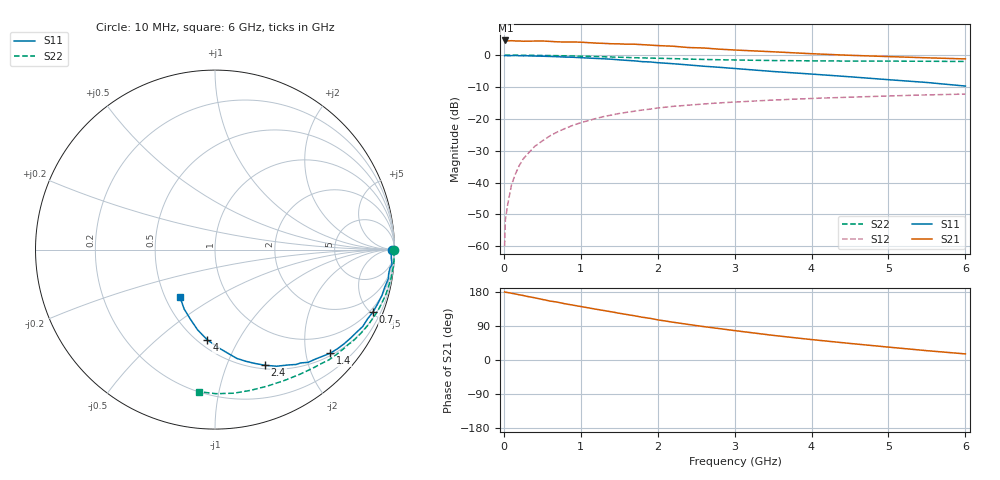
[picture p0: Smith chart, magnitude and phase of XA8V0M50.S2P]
! SIEMENS Discrete & RF Semiconductors
! BFY180
! Si NPN RF Bipolar Junction Transistor in MICRO-X
! VCE = 8 V  IC = 0.5 mA
! Common Emitter S-Parameters:  May  1997
# GHz  S  MA  R  50
!  f  S11  S21  S12  S22
! GHz  MAG  ANG  MAG  ANG  MAG  ANG  MAG  ANG
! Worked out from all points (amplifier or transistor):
!   36 points, 10 MHz to 6 GHz, reference 50 ohm
!   highest |S21| = 4.6 dB at 20 MHz (marker M1)
!   |S21| within 3 dB of that: start of sweep to 2.998 GHz
!   unconditionally stable (mu >= 1): nowhere
!   at 250 MHz: K = 0.05, MSG = 18.5 dB, |S12| = -32.7 dB
!   at 1.4 GHz: K = 0.37, MSG = 11.2 dB, |S12| = -18.8 dB
!   at 6 GHz: K = 1.00, MSG = 5.5 dB, |S12| = -12.2 dB
!   S11 on the Smith chart (normalised r, x): 10 MHz: open; 700 MHz: 0.78, -5.15; 1.4 GHz: 0.55, -2.51; 2.4 GHz: 0.54, -1.38; 4 GHz: 0.56, -0.75; 6 GHz: 0.60, -0.35
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0.01  0.9836 -0.2  1.684 179.5  0.001 90.7  0.9992 -0.2
0.02  0.9862 -0.5  1.704 178.9  0.0026 92.3  0.9999 -0.4
0.05  0.982 -1.5  1.676 178.1  0.0045 87.3  0.9994 -1.1
0.1  0.9838 -3.0  1.689 176.1  0.0092 88.3  0.9985 -2.2
0.15  0.99 -4.8  1.674 174.3  0.0136 86.3  0.9994 -3.4
0.25  0.9769 -7.8  1.657 170.3  0.0233 84.4  0.9984 -5.6
0.4  0.9687 -12.5  1.667 164.2  0.0368 80.6  0.9942 -8.9
0.6  0.9553 -18.5  1.647 155.6  0.0541 75.5  0.9867 -13.2
0.7  0.9463 -21.5  1.622 152.5  0.0627 73.0  0.9825 -15.4
0.9  0.9279 -27.5  1.614 144.7  0.0793 67.8  0.9714 -19.7
1.1  0.9018 -33.2  1.574 137.5  0.0939 63.7  0.9581 -23.8
1.4  0.8637 -41.9  1.513 127.1  0.1147 57.1  0.9373 -29.8
1.8  0.7916 -52.9  1.464 112.8  0.1378 49.4  0.9065 -37.2
2.2  0.7346 -62.2  1.383 99.7  0.1571 42.3  0.8838 -44.0
2.4  0.7023 -66.6  1.319 93.8  0.164 39.2  0.868 -47.1
2.6  0.6706 -70.9  1.297 88.1  0.1714 36.5  0.8579 -50.0
3  0.6181 -78.7  1.206 77.6  0.1836 31.1  0.8402 -55.8
3.5  0.5545 -86.8  1.131 65.0  0.1973 25.3  0.8246 -62.4
4  0.5052 -94.8  1.055 53.9  0.2091 20.1  0.8146 -69.0
4.5  0.4578 -102.2  0.996 43.7  0.2189 15.3  0.8089 -75.7
5.5  0.3727 -117.5  0.91 24.6  0.2379 5.9  0.8028 -89.6
6  0.3271 -126.8  0.874 16.1  0.2449 1.1  0.7966 -96.5
